FUNCTION_BLOCK FB_ProxyTcComIncrementModule EXTENDS FB_ProxyTcComModule
VAR_INPUT
END_VAR
VAR_OUTPUT
END_VAR
VAR
	_iThisProvider		: IIncrement;
END_VAR

METHOD FB_exit : BOOL
VAR_INPUT
	bInCopyCode : BOOL; // if TRUE, the exit method is called for exiting an instance that is copied afterwards (online change).
END_VAR
IF NOT bInCopyCode THEN
	FW_SafeRelease(pipUnk:= ADR(_iThisProvider));
END_IF
END_METHOD

METHOD FB_init : BOOL
VAR_INPUT
	bInitRetains 	: BOOL; // if TRUE, the retain variables are initialized (warm start / cold start)
	bInCopyCode 	: BOOL;  // if TRUE, the instance afterwards gets moved into the copy code (online change)
	IID				: IID;
END_VAR
ComQueryInterface(Super^._iProvider,TC_GLOBAL_IID_LIST.IID_IIncrement, ADR(_iThisProvider));
END_METHOD

PROPERTY ip : IIncrement
GET
ip	:= _iThisProvider;
END_GET
END_PROPERTY

END_FUNCTION_BLOCK
